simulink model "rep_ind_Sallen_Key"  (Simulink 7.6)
settings: Solver=ode15s  StartTime=0.0  StopTime=1e-3  RelTol=1e-3
InitFcn:
  | clc
libraries: fl_lib x8, nesl_utility x3

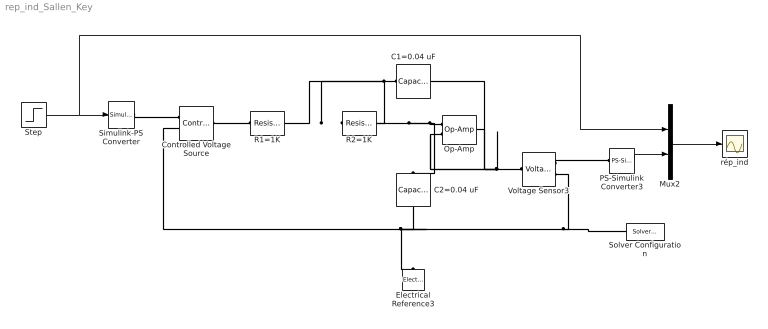
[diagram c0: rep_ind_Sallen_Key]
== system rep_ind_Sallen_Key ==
  C1=0.04 uF : fl_lib/Electrical/Electrical Elements/Capacitor  DialogController=NetworkEngine.DynNeDlgSource  SystemSampleTime=-1  c=0.04 uF  v0=0 V  r=1e-6 Ohm  g=0 1/Ohm  i_Log=off  v_Log=off  vc_Log=off  LocalVarNames=|i|v|vc  LocalVarDescs=|i|v|Internal variable for voltage across capacitor term  LocalVarLogging=[0 0 0]
  C2=0.04 uF : fl_lib/Electrical/Electrical Elements/Capacitor  DialogController=NetworkEngine.DynNeDlgSource  SystemSampleTime=-1  c=0.04 uF  v0=0 V  r=1e-6 Ohm  g=0 1/Ohm  i_Log=off  v_Log=off  vc_Log=off  LocalVarNames=|i|v|vc  LocalVarDescs=|i|v|Internal variable for voltage across capacitor term  LocalVarLogging=[0 0 0]
  Controlled Voltage Source : fl_lib/Electrical/Electrical Sources/Controlled Voltage Source  DialogController=NetworkEngine.DynNeDlgSource  SystemSampleTime=-1  i_Log=off  v_Log=off  LocalVarNames=|i|v  LocalVarDescs=|i|v  LocalVarLogging=[0 0]
  Electrical Reference3 : fl_lib/Electrical/Electrical Elements/Electrical Reference  DialogController=NetworkEngine.DynNeDlgSource  SystemSampleTime=-1  i_Log=off  LocalVarNames=|i  LocalVarDescs=|i  LocalVarLogging=[]
  Mux2 : Mux  Inputs=2
  Op-Amp : fl_lib/Electrical/Electrical Elements/Op-Amp  DialogController=NetworkEngine.DynNeDlgSource  SystemSampleTime=-1  i1_Log=off  v1_Log=off  outI_Log=off  LocalVarNames=|i1|v1|outI  LocalVarDescs=|i1|v1|outI  LocalVarLogging=[]
  PS-Simulink Converter3 : nesl_utility/PS-Simulink Converter  DialogController=NetworkEngine.DynNeUtilDlgSource  SystemSampleTime=-1  PhysicalDomain=network_engine_domain  LeftPortType=input  RightPortType=output  SubClassName=ps_output  Unit=1  AffineConversion=off
  R1=1K : fl_lib/Electrical/Electrical Elements/Resistor  DialogController=NetworkEngine.DynNeDlgSource  SystemSampleTime=-1  R=1 kOhm  i_Log=off  v_Log=off  LocalVarNames=|current|voltage|power  LocalVarDescs=|Resistor current (A)|Voltage across resistor (V)|Power (W)  LocalVarLogging=[0 0 0]
  R2=1K : fl_lib/Electrical/Electrical Elements/Resistor  DialogController=NetworkEngine.DynNeDlgSource  SystemSampleTime=-1  R=1 kOhm  i_Log=off  v_Log=off  LocalVarNames=|current|voltage|power  LocalVarDescs=|Resistor current (A)|Voltage across resistor (V)|Power (W)  LocalVarLogging=[0 0 0]
  Simulink-PS Converter : nesl_utility/Simulink-PS Converter  DialogController=NetworkEngine.DynNeUtilDlgSource  SystemSampleTime=-1  PhysicalDomain=network_engine_domain  LeftPortType=input  RightPortType=output  SubClassName=ps_input  Unit=1  AffineConversion=off  InputFilterTimeConstant=.001  UdotUserProvided=0
  Solver Configuration : nesl_utility/Solver Configuration  DialogController=NetworkEngine.DynNeUtilDlgSource  SystemSampleTime=-1  PhysicalDomain=network_engine_domain  LeftPortType=input  RightPortType=generic  SubClassName=solver  Accelerate=off  Profile=off  ResidualTolerance=1e-9  MaxNonlinIter=12  MaxModeIter=2  DoFixedCost=off  UseLocalSampling=off  DoDC=off  LinearAlgebra=Sparse  LocalSolverSampleTime=.001  LocalSolverChoice=NE_BACKWARD_EULER_ADVANCER  UseLocalSolver=off
  Step : Step  Time=0.0001  SampleTime=0
  Voltage Sensor3 : fl_lib/Electrical/Electrical Sensors/Voltage Sensor  DialogController=NetworkEngine.DynNeDlgSource  SystemSampleTime=-1  i1_Log=off  v1_Log=off  LocalVarNames=|i1|v1  LocalVarDescs=|i1|v1  LocalVarLogging=[]
  rép_ind : Scope
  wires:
  Step/1 -> Simulink-PS Converter/1, Mux2/1
  PS-Simulink Converter3/1 -> Mux2/2
  Mux2/1 -> rép_ind/1
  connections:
  Voltage Sensor3/RConn2 -- C2=0.04 uF/RConn1 -- Electrical Reference3/LConn1 -- Controlled Voltage Source/RConn2 -- Solver Configuration/RConn1
  Op-Amp/LConn1 -- R2=1K/RConn1 -- C2=0.04 uF/LConn1
  C1=0.04 uF/LConn1 -- R1=1K/RConn1 -- R2=1K/LConn1
  Op-Amp/LConn2 -- Voltage Sensor3/LConn1 -- Op-Amp/RConn1 -- C1=0.04 uF/RConn1
  Voltage Sensor3/RConn1 -- PS-Simulink Converter3/LConn1
  Simulink-PS Converter/RConn1 -- Controlled Voltage Source/RConn1
  Controlled Voltage Source/LConn1 -- R1=1K/LConn1
